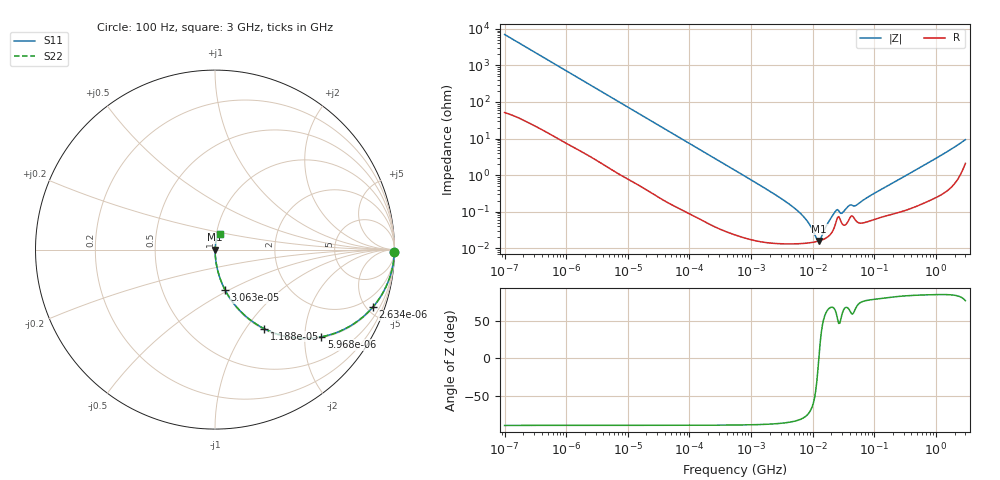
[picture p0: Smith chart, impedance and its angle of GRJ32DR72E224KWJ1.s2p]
!Murata Part Number: GRJ32DR72E224KWJ1
!These Parameters are Measured in Series Mode Connection
!Data Generated on Jun 19, 2026
!  o--ll--o
!Port1  Port2
!  o------o
!Operation Temp=25[degC], DC Bias Voltage=0[V]
!Freq. Start=100[Hz] Stop=3[GHz] 401[Steps]
# Hz S RI R 50
!Freq.(Hz) S11(Real) S11(Imag) S21(Real) S21(Imag) S12(Real) S12(Imag) S22(Real) S22(Imag)
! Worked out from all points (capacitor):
!   401 points, 100 Hz to 3 GHz, reference 50 ohm
!   read as one part in series: C = 227 nF near 109 Hz
!   lowest |Z| = 15.9 mohm at 12.68 MHz (marker M1)
!   series resonance near 12.56 MHz, so ESL is about 710 pH
!   S11 on the Smith chart (normalised r, x): 100 Hz: open; 2.634 kHz: 1.06, -5.44; 5.968 kHz: 1.03, -2.42; 11.88 kHz: 1.01, -1.22; 30.63 kHz: 1.01, -0.48; 3 GHz: 1.04, +0.18
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100  0.9997 -0.0143  0.000308 0.0143  0.000308 0.0143  0.9997 -0.0143
536  0.9936 -0.075  0.00643 0.075  0.00643 0.075  0.9936 -0.075
1788  0.9389 -0.2342  0.0611 0.2342  0.0611 0.2342  0.9389 -0.2342
2634  0.8784 -0.3214  0.1216 0.3214  0.1216 0.3214  0.8784 -0.3214
5968  0.5925 -0.4861  0.4075 0.4861  0.4075 0.4861  0.5925 -0.4861
11882  0.2731 -0.4401  0.7269 0.4401  0.7269 0.4401  0.2731 -0.4401
18274  0.1392 -0.3407  0.8608 0.3407  0.8608 0.3407  0.1392 -0.3407
30630  0.0558 -0.2242  0.9442 0.2242  0.9442 0.2242  0.0558 -0.2242
31977  0.0515 -0.2158  0.9485 0.2158  0.9485 0.2158  0.0515 -0.2158
102221  0.00599 -0.0714  0.994 0.0714  0.994 0.0714  0.00599 -0.0714
547723  0.000415 -0.0135  0.9996 0.0135  0.9996 0.0135  0.000415 -0.0135
4513443  0.000134 -0.00145  0.9999 0.00145  0.9999 0.00145  0.000134 -0.00145
7246509  0.000137 -0.000693  0.9999 0.000693  0.9999 0.000693  0.000137 -0.000693
9794414  0.000144 -0.000304  0.9999 0.000304  0.9999 0.000304  0.000144 -0.000304
1.163455e7  0.000153 -9.3e-05  0.9998 9.3e-05  0.9998 9.3e-05  0.000153 -9.3e-05
1.268047e7  0.000159 1.22e-05  0.9998 -1.22e-05  0.9998 -1.22e-05  0.000159 1.22e-05
2.316512e7  0.000439 0.000907  0.9996 -0.000907  0.9996 -0.000907  0.000439 0.000907
2.999103e7  0.000468 0.000794  0.9995 -0.000794  0.9995 -0.000794  0.000468 0.000794
3.882828e7  0.000612 0.00133  0.9994 -0.00133  0.9994 -0.00133  0.000612 0.00133
5.026954e7  0.000566 0.00137  0.9994 -0.00137  0.9994 -0.00137  0.000566 0.00137
1.751444e8  0.00084 0.00535  0.9992 -0.00535  0.9992 -0.00535  0.00084 0.00535
3e9  0.0281 0.0863  0.9719 -0.0863  0.9719 -0.0863  0.0281 0.0863
